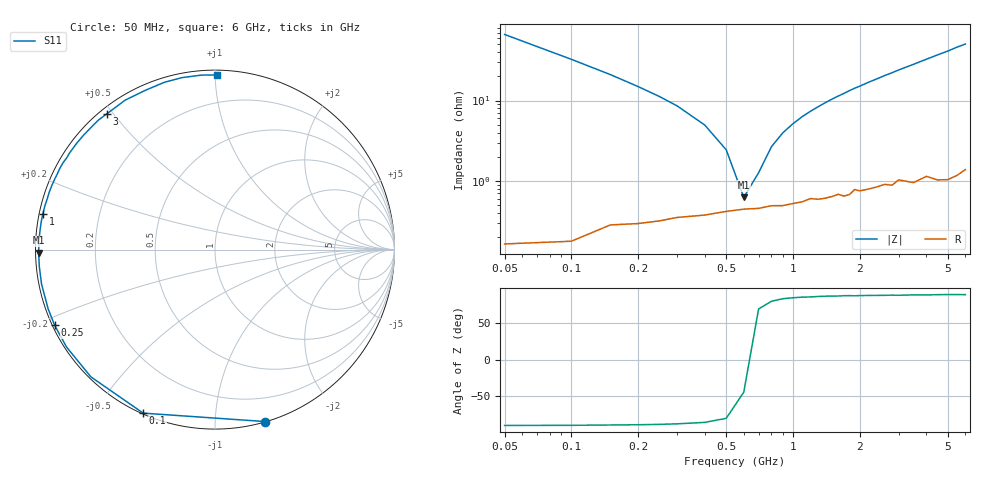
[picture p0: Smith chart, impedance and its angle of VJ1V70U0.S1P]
! Infineon Technologies  Discrete & RF Semiconductors
! BB 914
! Si Tuning Diode in SOT23
! VR = 1.75 V
! S-Parameters:  July  1999
# GHz  S  MA  R  50
!  f  S11
! GHz  MAG  ANG
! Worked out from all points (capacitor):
!   34 points, 50 MHz to 6 GHz, reference 50 ohm
!   read as one part to ground: C = 47.5 pF near 50 MHz
!   lowest |Z| = 623 mohm at 600 MHz (marker M1)
!   series resonance near 627 MHz, so ESL is about 1.4 nH
!   S11 on the Smith chart (normalised r, x): 50 MHz: 0.00, -1.33; 100 MHz: 0.00, -0.65; 250 MHz: 0.01, -0.22; 1 GHz: 0.01, +0.10; 3 GHz: 0.02, +0.48; 6 GHz: 0.03, +1.01
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0.05  0.9976 -73.8
0.1  0.995 -113.7
0.15  0.9905 -134.3
0.2  0.9893 -146.7
0.25  0.988 -154.7
0.3  0.9865 -160.5
0.4  0.9853 -168.7
0.5  0.9835 -174.5
0.6  0.9824 -179.0
0.7  0.982 177.3
0.8  0.9806 174.0
1  0.9796 168.3
1.1  0.9786 165.7
1.3  0.9773 161.0
1.6  0.9744 154.4
1.7  0.9759 152.4
1.9  0.9715 148.2
2.2  0.972 142.5
2.4  0.9708 139.0
2.6  0.9695 135.3
2.8  0.9709 132.1
3  0.9671 128.6
3.5  0.9716 121.0
4  0.9686 113.6
4.5  0.9739 106.8
5  0.9757 100.8
5.5  0.9751 94.4
6  0.9731 89.3
